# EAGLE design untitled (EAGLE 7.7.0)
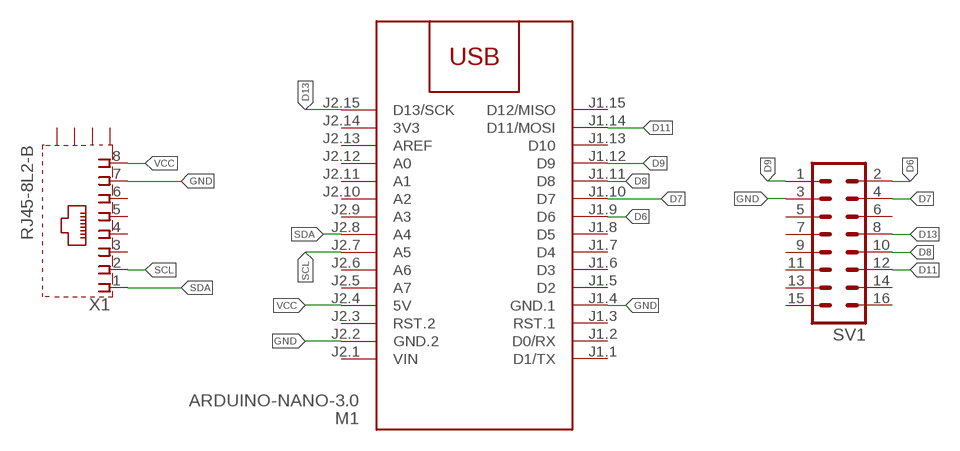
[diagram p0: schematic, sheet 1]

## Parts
M1  ARDUINO-NANO-3.0  [ARDUINO-NANO-3.0]
SV1  MA08-2  [MA08-2]
X1  RJ45-8L2-B  [RJ45-SHIELD2]

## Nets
D6: M1.J1.9(D6) SV1.2
D7: M1.J1.10(D7) SV1.4
D8: M1.J1.11(D8) SV1.10
D9: M1.J1.12(D9) SV1.1
D11: M1.J1.14(D11/MOSI) SV1.12
D13: M1.J2.15(D13/SCK) SV1.8
GND: M1.J1.4(GND.1) M1.J2.2(GND.2) SV1.3 X1.7
SCL: M1.J2.7(A5) X1.2
SDA: M1.J2.8(A4) X1.1
VCC: M1.J2.4(5V) X1.8
Unconnected: M1.J1.1(D1/TX) M1.J1.2(D0/RX) M1.J1.3(RST.1) M1.J1.5(D2) M1.J1.6(D3) M1.J1.7(D4) M1.J1.8(D5) M1.J1.13(D10) M1.J1.15(D12/MISO) M1.J2.3(RST.2) M1.J2.5(A7) M1.J2.6(A6) M1.J2.9(A3) M1.J2.10(A2) M1.J2.11(A1) M1.J2.12(A0) M1.J2.13(AREF) SV1.5 SV1.6 SV1.7 SV1.9 SV1.11 SV1.13 SV1.14 SV1.15 SV1.16 X1.3 X1.4 X1.5 X1.6 X1.S1(S) X1.S2(S) X1.S3(S) X1.S4(S)

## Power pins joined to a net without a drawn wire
3V3: M1.J2.14(3V3)
VIN: M1.J2.1(VIN)

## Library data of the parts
M1 = diy-modules:ARDUINO-NANO-3.0: Arduino Nano 3.0 and compatible devices More details available here: https://www.arduino.cc/en/Main/ArduinoBoardNano Click here to find device on ebay.com
SV1 = con-lstb:MA08-2: PIN HEADER; OC_FARNELL: unknown; OC_NEWARK: unknown
X1 = con-tycoelectronics:RJ45*2: RJ45 Low Profile Shield Type 2 For all RJ45 L, LC, LCT and X Series Models Source: www.tycoelectronics.com .. ENG_DS_1654001_1099_RJ_L_0507.pdf; MF: TYCO ELECTRONICS; MPN: RJ45-8L2-B; OC_FARNELL: unknown; OC_NEWARK: 52K3810

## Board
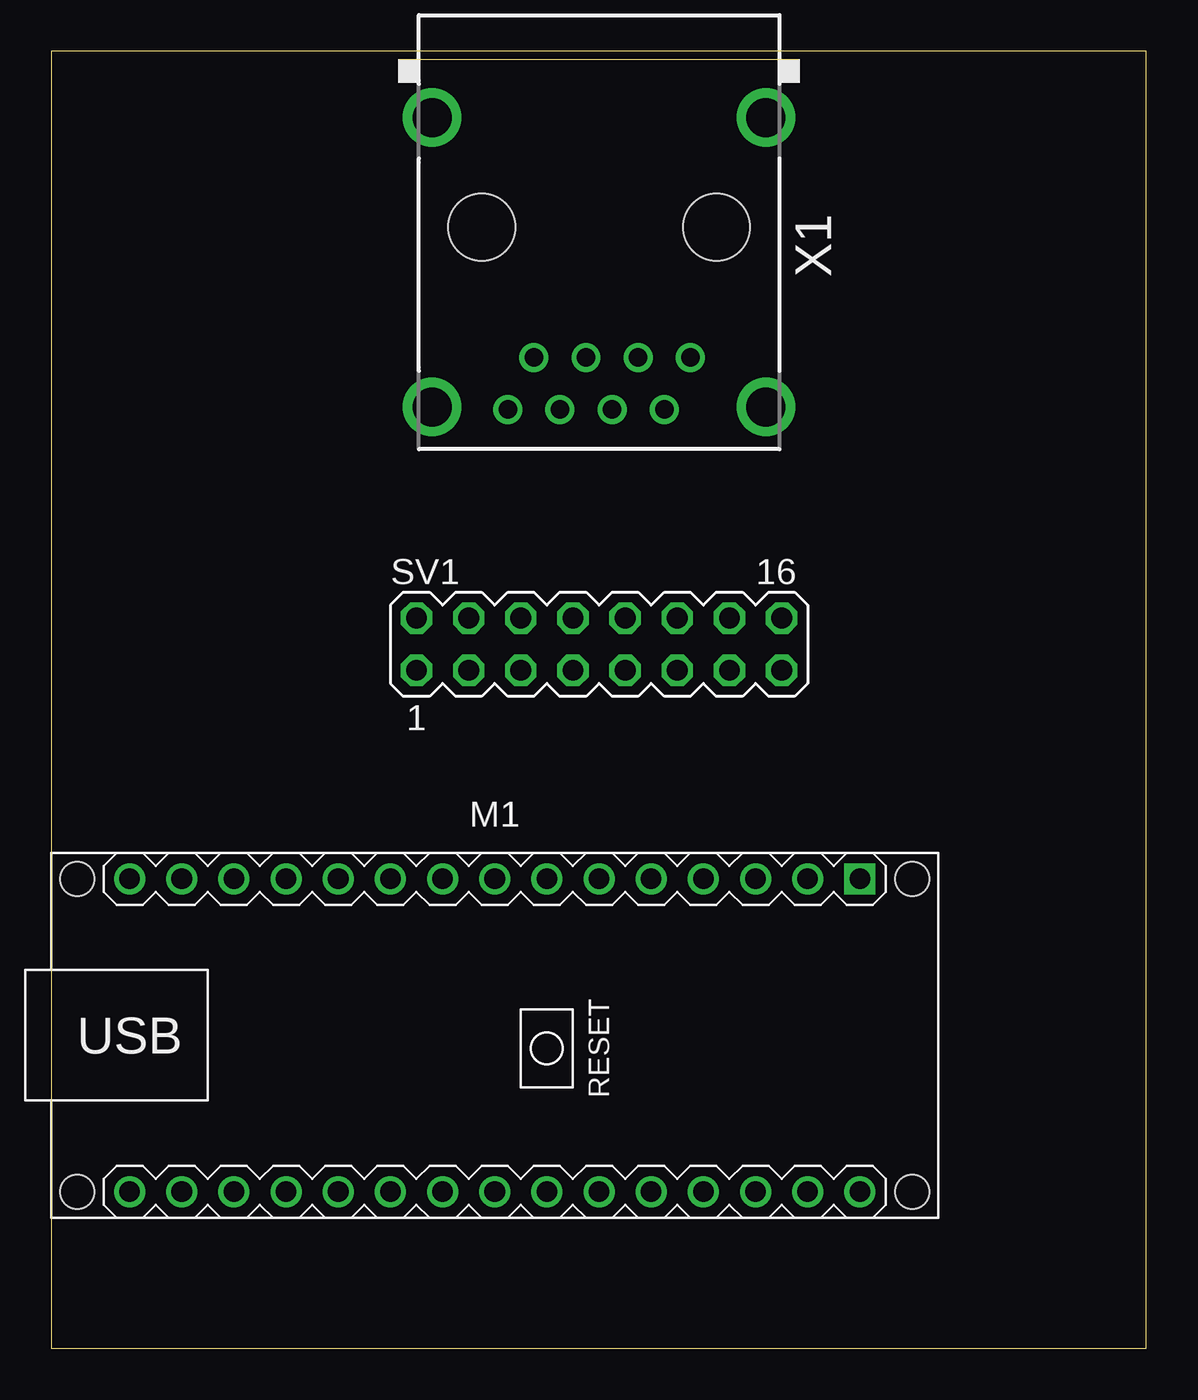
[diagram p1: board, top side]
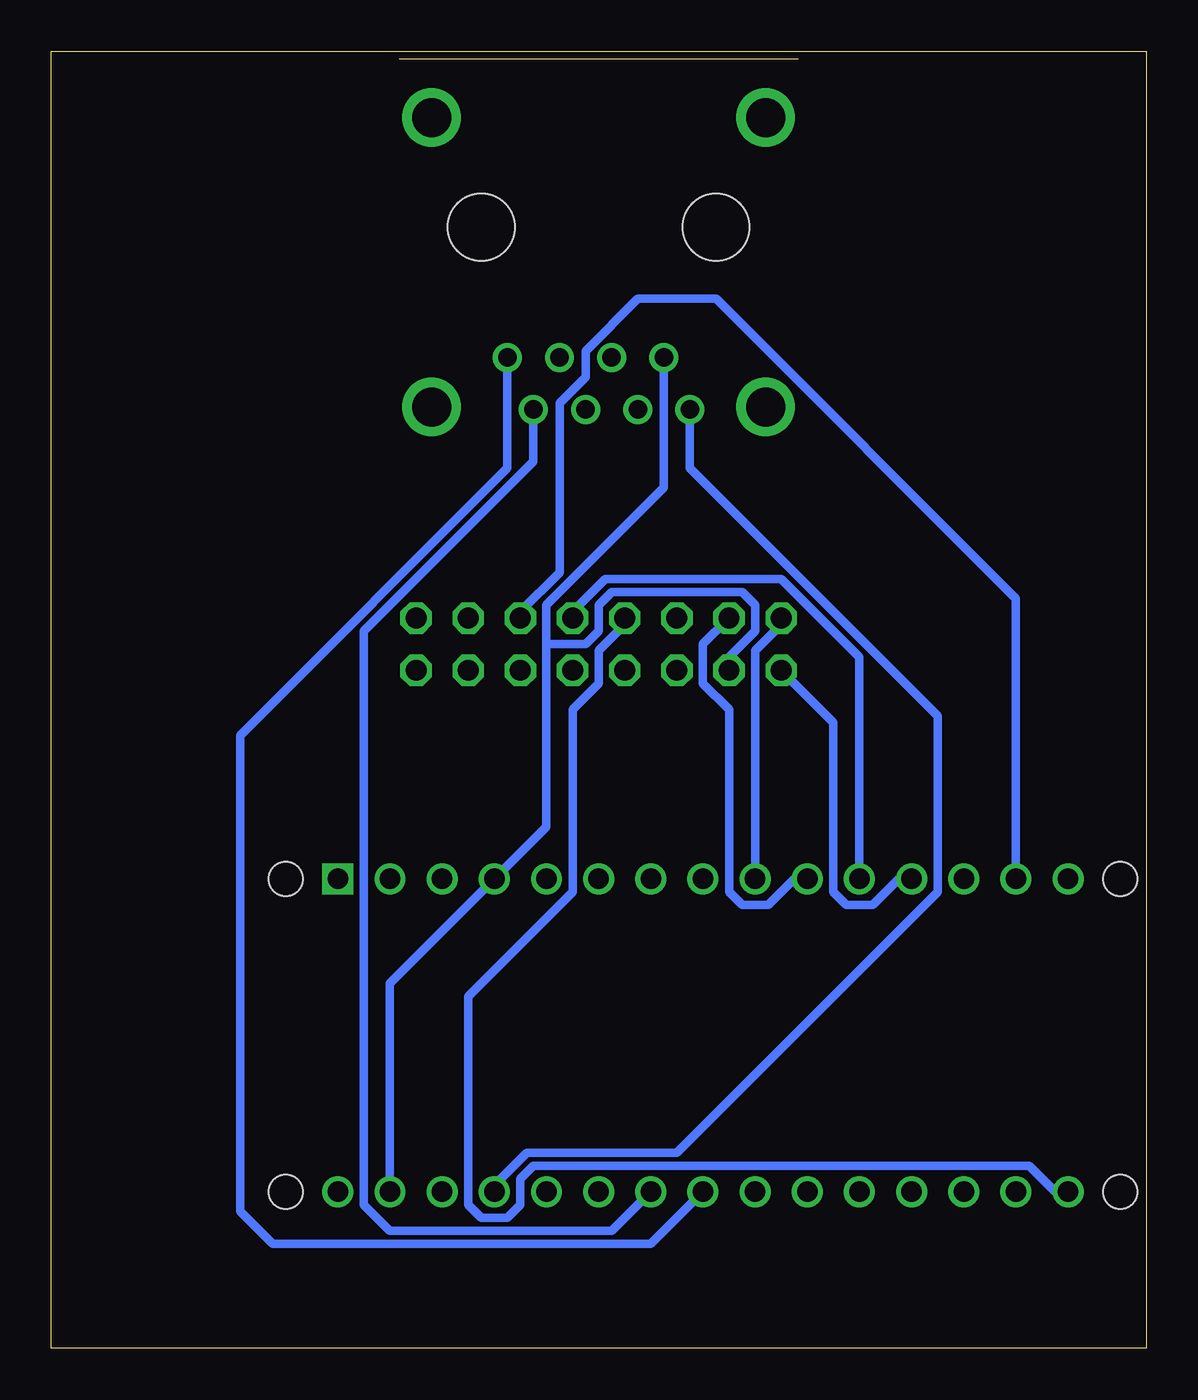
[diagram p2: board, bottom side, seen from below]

Size 53.32 x 63.17 mm. Coordinates in mm from the lower left corner, seen from the top.
Outline: 0,0 53.32,0 53.32,63.17 0,63.17 0,0
Copper layers (1*16): Top 0.035mm / dielectric 1.5mm / Bottom 0.035mm
Design rules "default *": minimum track width 16mil, minimum drill 24mil, track to track 8mil, track to pad 8mil, pad to pad 8mil, via to via 8mil, smd to smd 8mil, copper to edge 40mil, drill to drill 8mil, minimum pad ring 10mil, minimum via ring 8mil, stop-mask expansion 4mil, vias tented up to drill 0mil, thermal gap 10mil

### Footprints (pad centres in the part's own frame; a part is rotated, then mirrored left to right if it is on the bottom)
ARDUINO-NANO-3.0 = drill 1 square: J1.1 17.78,7.62 | drill 1: J1.2 15.24,7.62; J1.3 12.7,7.62; J1.4 10.16,7.62; J1.5 7.62,7.62; J1.6 5.08,7.62; J1.7 2.54,7.62; J1.8 0,7.62; J1.9 -2.54,7.62; J1.10 -5.08,7.62; J1.11 -7.62,7.62; J1.12 -10.16,7.62; J1.13 -12.7,7.62; J1.14 -15.24,7.62; J1.15 -17.78,7.62; J2.1 17.78,-7.62; J2.2 15.24,-7.62; J2.3 12.7,-7.62; J2.4 10.16,-7.62; J2.5 7.62,-7.62; J2.6 5.08,-7.62; J2.7 2.54,-7.62; J2.8 0,-7.62; J2.9 -2.54,-7.62; J2.10 -5.08,-7.62; J2.11 -7.62,-7.62; J2.12 -10.16,-7.62; J2.13 -12.7,-7.62; J2.14 -15.24,-7.62; J2.15 -17.78,-7.62 | hole 1.651: -20.32,7.62; -20.32,-7.62; 20.32,-7.62; 20.32,7.62
MA08-2 = drill 1.016 octagon: 1 -8.89,-1.27; 2 -8.89,1.27; 3 -6.35,-1.27; 4 -6.35,1.27; 5 -3.81,-1.27; 6 -3.81,1.27; 7 -1.27,-1.27; 8 -1.27,1.27; 9 1.27,-1.27; 10 1.27,1.27; 11 3.81,-1.27; 12 3.81,1.27; 13 6.35,-1.27; 14 6.35,1.27; 15 8.89,-1.27; 16 8.89,1.27
RJ45-SHIELD2 = drill 0.9 pad 1.4: 1 -4.445,6.35; 2 -3.175,8.89; 3 -1.905,6.35; 4 -0.635,8.89; 5 0.635,6.35; 6 1.905,8.89; 7 3.175,6.35; 8 4.445,8.89 | drill 1.9 pad 2.5: S1 -8.128,-5.33; S2 8.128,-5.33; S3 -8.128,8.76; S4 8.128,8.76 | hole 3.251: -5.715,0; 5.715,0

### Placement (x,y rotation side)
M1  21.59,15.24 0 top
SV1  26.67,34.29 0 top
X1  26.67,54.61 180 top

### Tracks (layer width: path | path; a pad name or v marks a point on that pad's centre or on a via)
D6
  Bottom 0.406: M1.J1.9 19.05,33.97 17.78,35.24 SV1.2
D7
  Bottom 0.406: M1.J1.10 17.14,22.86 18.41,21.59 19.68,21.59 20.32,22.23 20.32,31.11 21.59,32.38 21.59,34.29 SV1.4
D8
  Bottom 0.406: M1.J1.11 13.97,33.66 17.78,37.47 26.35,37.47 27.94,35.88 SV1.10
D9
  Bottom 0.406: M1.J1.12 12.06,22.86 13.34,21.59 14.61,21.59 15.24,22.23 15.24,30.48 SV1.1
D11
  Bottom 0.406: M1.J1.14 6.35,36.51 20.95,51.12 24.77,51.12 27.3,48.58 27.3,47.31 28.57,46.04 28.57,37.78 30.48,35.88 SV1.12
D13
  Bottom 0.406: M1.J2.15 4.45,7.62 5.71,8.89 29.84,8.89 30.48,8.26 30.48,6.99 31.11,6.35 32.38,6.35 33.02,6.99 33.02,17.14 27.94,22.23 27.94,31.11 26.67,32.38 26.67,33.97 25.4,35.24 SV1.8
GND
  Bottom 0.406: X1.7 23.5,41.91 29.21,36.2 29.21,34.29 | 29.21,34.29 29.21,25.4 M1.J1.4 36.83,17.78 M1.J2.2 | SV1.3 20.32,33.66 19.05,34.92 19.05,36.2 19.68,36.83 26.04,36.83 26.67,36.2 26.67,34.92 27.3,34.29 29.21,34.29
SCL
  Bottom 0.406: X1.2 29.84,43.18 38.1,34.92 38.1,6.99 36.83,5.71 26.04,5.71 M1.J2.7
SDA
  Bottom 0.406: X1.1 31.11,42.86 44.13,29.84 44.13,6.67 42.55,5.08 24.13,5.08 M1.J2.8
VCC
  Bottom 0.406: X1.8 22.23,42.86 10.16,30.8 10.16,22.23 22.86,9.53 30.16,9.53 31.75,7.94 M1.J2.4

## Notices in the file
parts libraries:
diy-modules: Released under the Creative Commons Attribution 4.0 International License: http://creativecommons.org/licenses/by/4.0
